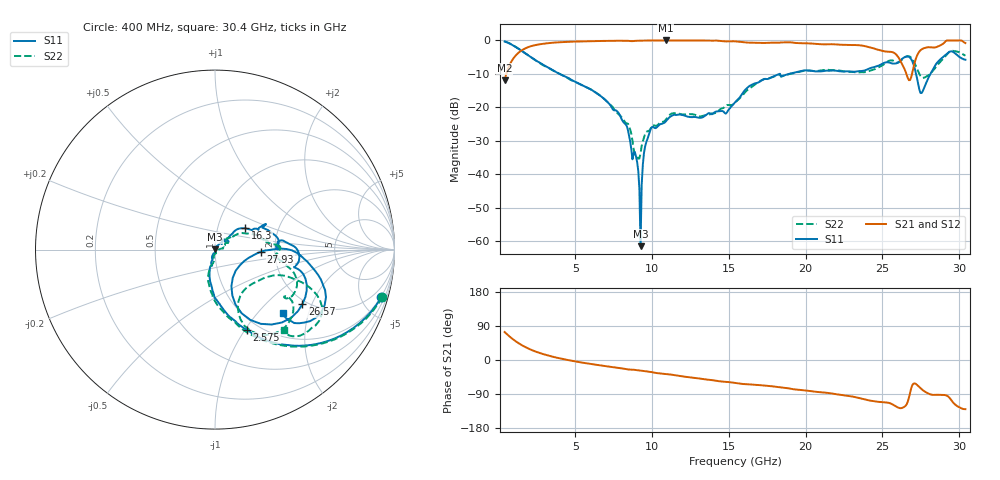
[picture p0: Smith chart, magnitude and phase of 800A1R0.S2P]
!  American Technical Ceramics  Date:  9/12/2007
!  One Norden Lane
!  Huntington Station,  NY.  11746-2102
!  Tel:  (631) 622-4700  Fax:  (631) 622-4748
!  Part Number  800A1R0  Mounting Orientation: Vertical
!  Description: Ultra Low ESR Microwave capacitors
!  Application: Coupling, Bypass, Tuning, DC Block
!  Filters, Matching
# GHZ S DB R 50
! Freq  |S11|  S11 Ph  |S21|  S21 Ph  |S12|  S12 Ph  |S22|  S22 Ph
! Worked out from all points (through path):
!   401 points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, 400 MHz to 30.4 GHz, reference 50 ohm
!   highest |S21| = -0.01 dB at 10.9 GHz (marker M1); lowest = -11.9 dB at 400 MHz (marker M2)
!   group delay of S21, straight-line fit = 13.8 ps
!   lowest |S11| = -61.4 dB at 9.25 GHz (marker M3), VSWR 1.00, Z = 50 + j0.0701 ohm
!   |S11| at or under -10 dB: 3.972 GHz to 18.29 GHz (14.32 GHz wide, 129 % of centre); 18.33 GHz to 18.9 GHz (570.1 MHz wide, 3.06 % of centre); 27.19 GHz to 28.12 GHz (936.1 MHz wide, 3.38 % of centre)
!   |S22| runs from -35.3 to -0.3 dB; largest |S21 - S12| = 0.0033
!   S11 on the Smith chart (normalised r, x): 400 MHz: 0.93, -6.98; 2.575 GHz: 0.88, -1.02; 16.3 GHz: 1.35, +0.34; 26.57 GHz: 1.89, -1.71; 27.93 GHz: 1.68, -0.04; 30.4 GHz: 1.43, -1.37
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0.4  -0.32 -16.0  -11.93 73.8  -11.92 73.7  -0.27 -15.9
1.3  -2.48 -45.0  -3.70 44.6  -3.69 44.5  -2.44 -45.3
2.575  -6.35 -68.3  -1.24 20.0  -1.24 20.0  -6.41 -70.3
5.425  -13.32 -94.5  -0.30 -6.8  -0.30 -6.8  -13.31 -97.6
8.275  -25.02 -103.6  -0.07 -23.6  -0.07 -23.7  -24.61 -93.1
8.95  -34.54 -80.7  -0.11 -26.5  -0.11 -26.5  -34.26 -60.2
9.1  -38.81 -85.0  -0.10 -27.4  -0.11 -27.4  -35.30 -37.3
9.25  -61.40 55.3  -0.09 -28.0  -0.09 -28.0  -33.76 -0.4
9.7  -29.42 53.7  -0.01 -30.5  -0.01 -30.5  -27.08 6.9
10.45  -25.29 45.7  -0.01 -35.2  -0.01 -35.2  -24.87 20.9
10.9  -24.12 51.0  -0.01 -37.1  -0.01 -37.1  -23.64 30.3
15.4  -18.47 42.7  -0.27 -60.7  -0.28 -60.6  -18.59 36.2
16.3  -13.74 35.4  -0.66 -64.2  -0.66 -64.2  -14.47 28.7
20.425  -9.12 3.5  -0.95 -82.7  -0.94 -82.7  -9.05 1.2
25.45  -6.62 -9.5  -3.36 -113.5  -3.36 -113.5  -6.04 -23.6
26.575  -4.82 -32.0  -10.21 -117.1  -10.24 -116.8  -4.77 -44.4
27.175  -9.73 -69.5  -5.45 -63.2  -5.46 -63.1  -7.61 -69.9
27.55  -15.70 -32.0  -2.68 -77.2  -2.69 -77.1  -11.02 -56.6
27.925  -11.86 -2.7  -2.06 -87.2  -2.07 -87.1  -10.59 -36.3
29.275  -3.69 -20.3  -0.01 -96.2  -0.01 -96.1  -3.76 -25.7
29.875  -4.40 -42.8  -0.01 -121.9  -0.01 -121.8  -3.35 -44.1
30.4  -5.76 -43.0  -0.79 -129.8  -0.78 -129.7  -4.55 -49.3
